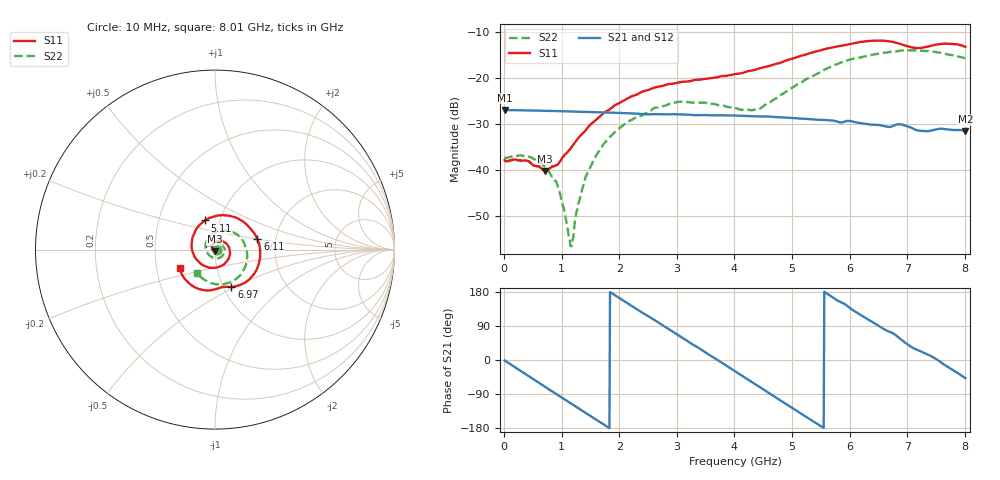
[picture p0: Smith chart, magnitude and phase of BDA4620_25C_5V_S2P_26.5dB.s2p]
!Agilent Technologies,E5071B,MY42404982,A.09.10
!Date: Wed May 06 09:04:13 2026
!Data & Calibration Information:
!Freq	S11:SOLT2(ON)	S21:SOLT2(ON)	S12:SOLT2(ON)	S22:SOLT2(ON)
# Hz S RI R 50
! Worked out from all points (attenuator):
!   801 points, 10 MHz to 8.01 GHz, reference 50 ohm
!   highest |S21| = -26.88 dB at 10 MHz (marker M1); lowest = -31.5 dB at 8.01 GHz (marker M2)
!   lowest |S11| = -40.2 dB at 710 MHz (marker M3), VSWR 1.02, Z = 49.8 - j0.961 ohm
!   |S11| at or under -10 dB: start of sweep to end of sweep
!   |S22| runs from -56.5 to -13.9 dB; largest |S21 - S12| = 0.00023
!   S11 on the Smith chart (normalised r, x): 10 MHz: 1.03, -0.00; 5.11 GHz: 0.85, +0.28; 6.11 GHz: 1.60, +0.20; 6.97 GHz: 1.09, -0.48; 8.01 GHz: 0.66, -0.14
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1e7  0.0128 -0.000792  0.0453 -0.000928  0.0453 -0.00101  0.0134 -0.000457
4.4e8  0.00812 -0.00929  0.0322 -0.0309  0.0322 -0.0309  0.0132 -0.00475
7.1e8  -0.00165 -0.00964  0.0148 -0.0417  0.0148 -0.0418  0.00854 -0.00673
9.3e8  -0.0104 -0.00491  -0.00155 -0.0439  -0.00165 -0.0439  0.00357 -0.00578
1.16e9  -0.0163 0.00609  -0.0181 -0.0395  -0.0182 -0.0396  -0.00127 -0.000779
1.19e9  -0.0167 0.00786  -0.0201 -0.0385  -0.0202 -0.0385  -0.00176 6.35e-05
1.26e9  -0.0173 0.0123  -0.0244 -0.0357  -0.0245 -0.0357  -0.00279 0.00224
1.35e9  -0.0169 0.0178  -0.0295 -0.0315  -0.0296 -0.0315  -0.00326 0.00495
1.53e9  -0.0123 0.03  -0.0373 -0.021  -0.0374 -0.021  -0.00304 0.0115
1.77e9  0.00188 0.0433  -0.0421 -0.00446  -0.0422 -0.00446  0.00108 0.0205
2.15e9  0.0377 0.0475  -0.0358 0.0214  -0.0358 0.0214  0.0173 0.029
2.68e9  0.0808 0.00573  -0.0062 0.0401  -0.00616 0.0402  0.0443 0.0191
3.08e9  0.0754 -0.0511  0.02 0.0351  0.0202 0.0351  0.055 -0.00758
4.01e9  -0.0734 -0.0829  0.0341 -0.0195  0.0341 -0.0195  -0.0106 -0.0462
4.43e9  -0.1275 -0.00196  0.0129 -0.0362  0.0129 -0.0362  -0.045 -0.0115
5.11e9  -0.0558 0.1623  -0.0268 -0.025  -0.0268 -0.025  -0.0168 0.0855
5.35e9  0.016 0.1899  -0.0336 -0.0121  -0.0336 -0.0122  0.0233 0.1021
6.11e9  0.2359 0.0589  -0.0196 0.0267  -0.0197 0.0268  0.1605 0.0393
6.68e9  0.1892 -0.1676  0.0075 0.0285  0.00754 0.0286  0.1697 -0.0897
6.97e9  0.091 -0.2073  0.0215 0.0215  0.0217 0.0216  0.1306 -0.1523
7.59e9  -0.0789 -0.2227  0.028 -0.00329  0.028 -0.00333  -0.0197 -0.1875
8.01e9  -0.1955 -0.1005  0.0178 -0.0197  0.0179 -0.0197  -0.1028 -0.1282
